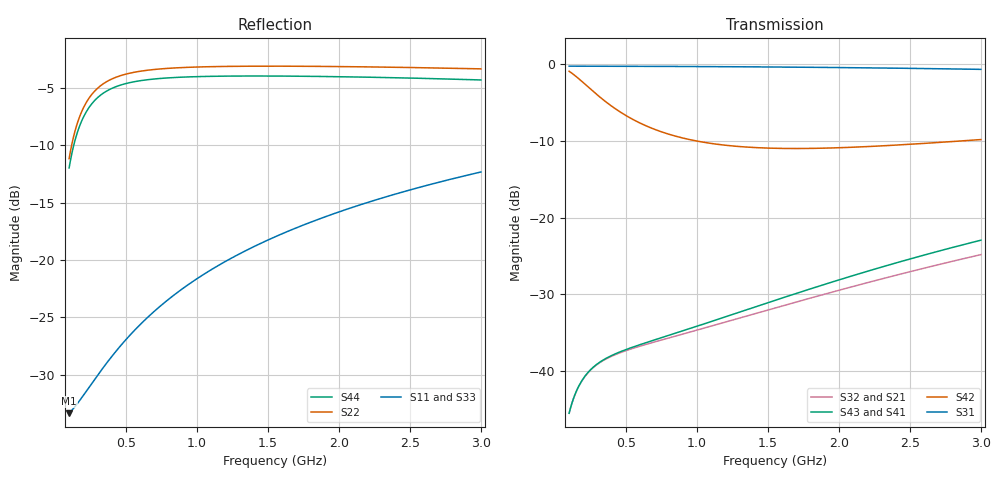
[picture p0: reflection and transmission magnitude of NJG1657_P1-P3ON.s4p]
! NJG1657MD7(1bit control high power DPDT switch) S-parameter
! VDD=2.85V, VCTL(H)=2.6V, VCTL(L)=0V
! P1-P3 ON mode
! Port1...P1, Port2...P2, Port3...P3, Port4...P4
# hz S ma R 50
! 4 Port Network Data from SP1.SP block
! freq  magS11  angS11  magS12  angS12  magS13  angS13  magS14  angS14
!  magS21  angS21  magS22  angS22  magS23  angS23  magS24  angS24
!  magS31  angS31  magS32  angS32  magS33  angS33  magS34  angS34
!  magS41  angS41  magS42  angS42  magS43  angS43  magS44  angS44
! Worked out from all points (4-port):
!   291 points, 100 MHz to 3 GHz, reference 50 ohm
!   strongest paths, dB at 100 MHz, 820 MHz, 1.55 GHz, 2.28 GHz, 3 GHz:
!     S31: -0.2, -0.3, -0.3, -0.5, -0.6
!     S42: -0.9, -9.2, -11.0, -10.7, -9.8
!     S43: -45.6, -35.3, -30.8, -26.6, -23.0
!     S41: -45.6, -35.3, -30.9, -26.7, -23.1
!     S32: -45.6, -35.6, -31.8, -28.1, -24.8
!     S21: -45.6, -35.7, -31.9, -28.2, -24.9
!   lowest |S11| = -33.4 dB at 100 MHz (marker M1), VSWR 1.04, Z = 52 - j0.898 ohm
!   |S11| at or under -10 dB: start of sweep to end of sweep
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1e8  0.02147 -23.7  0.005244 66.2  0.9735 -1.2  0.005263 67.0
     0.005244 66.2  0.2765 -109.7  0.005262 66.3  0.9016 -17.1
     0.9735 -1.2  0.005262 66.3  0.02161 -23.6  0.005273 67.0
     0.005263 67.0  0.9016 -17.1  0.005273 67.0  0.252 -109.9
1.7e8  0.02422 -37.0  0.007933 59.7  0.9733 -2.0  0.00797 61.0
       0.007933 59.7  0.415 -124.8  0.007961 59.8  0.8033 -26.0
       0.9733 -2.0  0.007961 59.8  0.0244 -36.8  0.007985 61.1
       0.00797 61.0  0.8033 -26.0  0.007985 61.1  0.3779 -125.6
2.8e8  0.03017 -52.3  0.01062 52.6  0.9729 -3.3  0.0107 54.7
       0.01062 52.6  0.5447 -141.1  0.01066 52.8  0.6535 -34.2
       0.9729 -3.3  0.01066 52.8  0.03046 -51.9  0.01072 54.9
       0.0107 54.7  0.6535 -34.2  0.01072 54.9  0.4959 -142.6
4.6e8  0.04213 -67.8  0.01304 48.9  0.9721 -5.5  0.01325 52.4
       0.01304 48.9  0.6355 -156.8  0.01309 49.3  0.4886 -38.1
       0.9721 -5.5  0.01309 49.3  0.0426 -66.9  0.01328 52.6
       0.01325 52.4  0.4886 -38.1  0.01328 52.6  0.5781 -159.4
7.1e8  0.06054 -80.2  0.01541 51.0  0.9706 -8.5  0.01592 56.2
       0.01541 51.0  0.6778 -168.9  0.01547 51.6  0.3742 -35.7
       0.9706 -8.5  0.01547 51.6  0.06128 -78.7  0.01596 56.5
       0.01592 56.2  0.3742 -35.7  0.01596 56.5  0.616 -173.0
1.61e9  0.131 -103.2  0.02646 64.9  0.9604 -19.2  0.02983 73.0
        0.02646 64.9  0.6994 170.2  0.02658 66.3  0.2825 -19.6
        0.9604 -19.2  0.02658 66.3  0.1327 -99.5  0.03 73.7
        0.02983 73.0  0.2825 -19.6  0.03 73.7  0.6333 160.9
3e9  0.2419 -127.1  0.05695 67.6  0.9279 -36.0  0.07012 74.1
     0.05695 67.6  0.681 150.3  0.05723 70.2  0.3229 -12.2
     0.9279 -36.0  0.05723 70.2  0.2448 -120.2  0.07109 75.5
     0.07012 74.1  0.3229 -12.2  0.07109 75.5  0.6091 133.1
